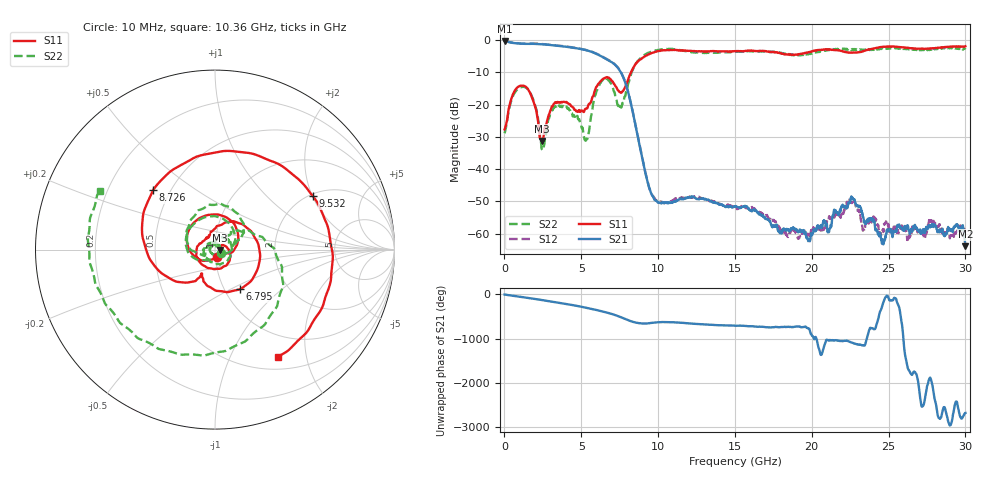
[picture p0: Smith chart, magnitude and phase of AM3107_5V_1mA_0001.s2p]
# Hz S DB R 50.0
!freq dBS11 angS11 dBS21 angS21 dBS12 angS12 dBS22 angS22
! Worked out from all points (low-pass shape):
!   1601 points, 10 MHz to 30 GHz, reference 50 ohm
!   highest |S21| = -0.26 dB at 10 MHz (marker M1); lowest = -63.9 dB at 30 GHz (marker M2)
!   |S21| within 3 dB of the highest: start of sweep to 5.411 GHz
!   lowest |S11| = -31.3 dB at 2.447 GHz (marker M3), VSWR 1.06, Z = 52.8 - j0.235 ohm
!   |S11| at or under -10 dB: start of sweep to 8.237 GHz
!   |S22| runs from -34.1 to -2.2 dB; largest |S21 - S12| = 0.016
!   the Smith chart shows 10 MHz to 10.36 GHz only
!   S11 on the Smith chart (normalised r, x): 10 MHz: 1.02, -0.08; 6.795 GHz: 1.18, -0.56; 8.726 GHz: 0.40, +0.35; 9.532 GHz: 2.07, +2.01; 10.36 GHz: 0.67, -1.54
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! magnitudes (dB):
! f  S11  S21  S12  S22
! 10 MHz  -27.7  -0.3  -0.1  -28.9
! 591.1 MHz  -16.4  -0.9  -0.8  -17.0
! 1.341 GHz  -14.4  -1.2  -1.1  -14.6
! 1.978 GHz  -20.4  -1.2  -1.1  -20.0
! 2.447 GHz  -31.3  -1.3  -1.2  -33.9
! 3.328 GHz  -19.3  -1.7  -1.6  -20.4
! 5.015 GHz  -21.9  -2.8  -2.7  -27.0
! 5.352 GHz  -21.3  -3.2  -3.1  -30.7
! 6.008 GHz  -14.4  -4.3  -4.2  -15.7
! 6.795 GHz  -11.7  -6.3  -6.2  -12.5
! 7.601 GHz  -16.4  -10.2  -10.1  -20.9
! 8.726 GHz  -6.4  -31.1  -30.9  -6.3
! 9.532 GHz  -4.1  -47.3  -47.1  -3.7
! 10.02 GHz  -3.4  -50.4  -50.0  -3.1
! 10.36 GHz  -3.2  -50.4  -50.5  -2.9
! 15.01 GHz  -3.5  -51.7  -51.7  -3.5
! 20.01 GHz  -3.5  -60.5  -58.0  -4.1
! 22.65 GHz  -3.9  -49.0  -49.3  -2.9
! 23.35 GHz  -3.5  -54.8  -58.9  -3.0
! 25.01 GHz  -2.0  -59.4  -58.7  -2.6
! 29.42 GHz  -1.9  -57.1  -59.5  -2.4
! 30 GHz  -1.9  -63.9  -59.4  -2.4
